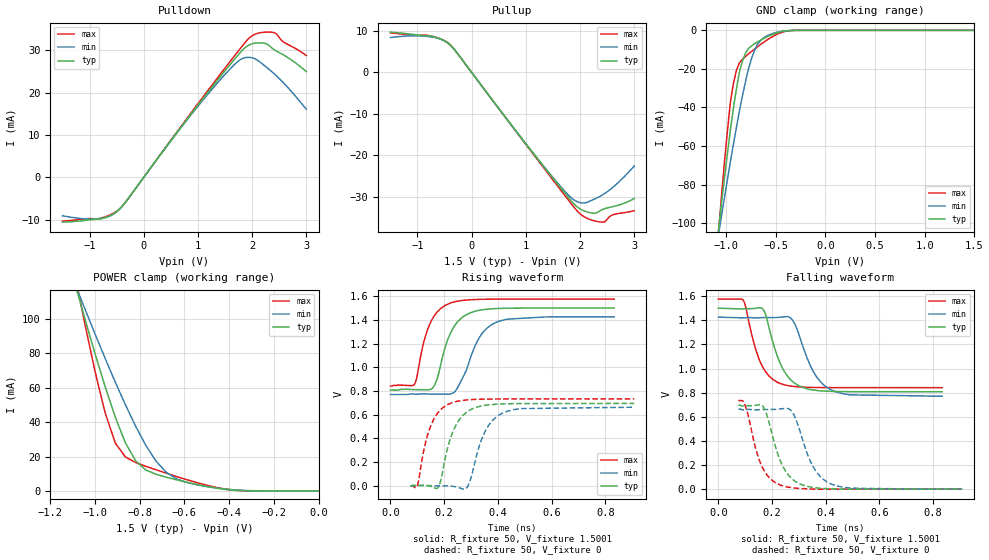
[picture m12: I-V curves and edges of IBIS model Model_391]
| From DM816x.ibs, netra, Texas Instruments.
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| Model based on original model for BSHTLTCSCDDVGPBFZ
|   Sub model FASTEST_7MA_5PER_N_1P5
[model]   Model_391
|[Description]  1.5V-3-STATE-X-FASTEST, 7MA, +-5%
|[Input Load]
|[Output Drive] FASTEST, 7MA
|Voltage   1.5V
|Mode   3-STATE
Model_type   3-state
Polarity   Non-Inverting
Enable   Active-Low
Cref =  15.0000pF
Rref =  100.0000M
Vref =  0V
Vmeas =  0.75005
C_comp   1.5249p   1.4275p   1.6205p
[Model Spec]
[Temperature Range]   25   125   -40
[Voltage Range]   1.5   1.425   1.575
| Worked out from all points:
|   slope of the pulldown table from 0 to 0.225 V, typ, clamps not added: 57.5 ohm
|   slope of the pullup table from 0 to 0.225 V, typ, clamps not added: 57.5 ohm
|   GND clamp passes 1 mA (typ) near -0.47 V on its own axis
|   POWER clamp passes 1 mA (typ) near -0.42 V on its own axis
|   rising waveform, R_fixture 50, V_fixture 1.5001: 20-80 % time 63.2ps typ, 77.9ps min, 57.5ps max; typ from 0.808 V to 1.5 V
|   rising waveform, R_fixture 50, V_fixture 0: 20-80 % time 60.1ps typ, 65.2ps min, 55.9ps max; typ from 0 V to 0.695 V
|   falling waveform, R_fixture 50, V_fixture 1.5001: 20-80 % time 68.2ps typ, 77.9ps min, 62.1ps max; typ from 1.5 V to 0.807 V
|   falling waveform, R_fixture 50, V_fixture 0: 20-80 % time 65.3ps typ, 72.4ps min, 59ps max; typ from 0.696 V to 0 V
[POWER_clamp]
-1.5V     321.7mA    260.6mA    415.9mA
-1.076V   114.2mA    115.8mA    116.9mA
-1.061V   107.2mA    110.9mA    107.1mA
-954.6mV  60.59mA    77.06mA    45.35mA
-909.2mV  42.85mA    63.21mA    27.81mA
-863.7mV  27.9mA     49.99mA    19.69mA
-818.2mV  17.49mA    37.63mA    16.52mA
-772.8mV  12.19mA    26.53mA    14.33mA
-681.9mV  7.985mA    10.89mA    10.33mA
-590.9mV  5.094mA    4.955mA    6.6mA
-363.7mV  298.5uA    465.2uA    297.6uA
0V        1.518nA    24.08nA    367.8pA
[Pulldown]
-1.5V     -10.59mA   -9.07mA    -10.35mA
-863.7mV  -9.876mA   -9.778mA   -9.846mA
-500mV    -8.072mA   -8.154mA   -8.005mA
-318.2mV  -5.535mA   -5.556mA   -5.589mA
1.046V    17.79mA    17.48mA    18.14mA
1.591V    26.54mA    25.51mA    27.28mA
1.818V    29.96mA    28.01mA    30.98mA
1.955V    31.28mA    28.29mA    32.97mA
2.091V    31.69mA    27.68mA    33.92mA
2.273V    31.43mA    25.88mA    34.25mA
2.364V    30.5mA     24.91mA    34.22mA
3V        24.94mA    16.04mA    28.71mA
[Pullup]
-1.5V     9.77mA     8.45mA     9.58mA
-818.2mV  8.911mA    8.699mA    9.007mA
-590.9mV  8.189mA    8.133mA    8.203mA
-409.1mV  6.819mA    6.785mA    6.878mA
1.227V    -21.03mA   -21.02mA   -21.31mA
1.727V    -29.3mA    -28.85mA   -29.87mA
1.909V    -32.06mA   -30.99mA   -32.91mA
2.046V    -33.31mA   -31.56mA   -34.63mA
2.227V    -34.01mA   -30.83mA   -35.73mA
2.409V    -33.14mA   -29.62mA   -36.19mA
2.591V    -32.48mA   -27.92mA   -34.46mA
3V        -30.47mA   -22.61mA   -33.42mA
[GND_clamp]
-1.5V     -310.1mA   -250.5mA   -402.5mA
-1.076V   -103.6mA   -106.2mA   -105.2mA
-1.046V   -89.81mA   -96.36mA   -86.02mA
-954.6mV  -51.22mA   -67.87mA   -36.88mA
-924.3mV  -40.08mA   -58.86mA   -27.29mA
-863.7mV  -21.24mA   -41.56mA   -16.73mA
-833.4mV  -15.8mA    -33.75mA   -15.03mA
-772.8mV  -9.345mA   -19.75mA   -12.19mA
-712.2mV  -6.928mA   -10.35mA   -9.704mA
-621.3mV  -4.261mA   -3.896mA   -6.225mA
-409.1mV  -337.1uA   -289.1uA   -618.9uA
1.5V      1.518nA    257.2nA    299pA
[Ramp]
dV/dt_f   0.557592/0.10776819n   0.527888/0.12384948n   0.58756/97.222028p
dV/dt_r   0.573716/97.043568p  0.5525896/0.10588527n  0.5985464/88.899722p
R_load = 50
[Rising Waveform]
R_fixture = 50
V_fixture = 1.5001
V_fixture_min = 1.425
V_fixture_max = 1.575
0s        808.1mV    770.8mV    842.1mV
90.36ps   811.7mV    773.9mV    860.2mV
129.6ps   810.4mV    775.7mV    1.256V
157ps     824.8mV    774mV      1.41V
173.9ps   901.6mV    774.4mV    1.465V
224.8ps   1.293V     776.1mV    1.543V
266.9ps   1.42V      901mV      1.563V
327.9ps   1.479V     1.238V     1.572V
388.6ps   1.495V     1.374V     1.574V
833.3ps   1.5V       1.425V     1.575V
[Rising Waveform]
R_fixture = 50
V_fixture = 0
V_fixture_min = 0
V_fixture_max = 0
74.7ps    0V         0V         0V
99.62ps   2.847mV    2.73mV     0V
137.1ps   0V         4.126mV    418.4mV
177.7ps   -14.03mV   0V         618.8mV
230.7ps   445.2mV    -2.995mV   702.7mV
288.4ps   629.6mV    -2.255mV   725.6mV
330.3ps   668.7mV    332.5mV    730.5mV
353.8ps   679.6mV    465.3mV    731.7mV
417.4ps   691.3mV    613.6mV    733.1mV
908ps     695.3mV    663.5mV    733.6mV
[Falling Waveform]
R_fixture = 50
V_fixture = 1.5001
V_fixture_min = 1.425
V_fixture_max = 1.575
0s        1.5V       1.426V     1.576V
92.77ps   1.495V     1.419V     1.566V
137.8ps   1.499V     1.419V     1.17V
165.5ps   1.494V     1.422V     1.012V
222.4ps   1.088V     1.424V     883.1mV
276ps     893.5mV    1.403V     852.7mV
350.3ps   823.4mV    989.7mV    843.2mV
421.4ps   810.6mV    821.4mV    841.8mV
491.7ps   808mV      781.6mV    841.5mV
833.3ps   807.4mV    770.2mV    841.4mV
[Falling Waveform]
R_fixture = 50
V_fixture = 0
V_fixture_min = 0
V_fixture_max = 0
74.7ps    695.7mV    664.1mV    734.5mV
99.89ps   690.4mV    659.1mV    692.8mV
140.8ps   695.8mV    657.5mV    323.8mV
165.7ps   688.8mV    660.1mV    175mV
183.4ps   594.9mV    660.5mV    112.1mV
231ps     235mV      665.3mV    33.48mV
275.1ps   84.31mV    640.1mV    11.61mV
351.2ps   14.37mV    193.6mV    0V
422.7ps   3.003mV    40.38mV    0V
908ps     0V         0V         0V
